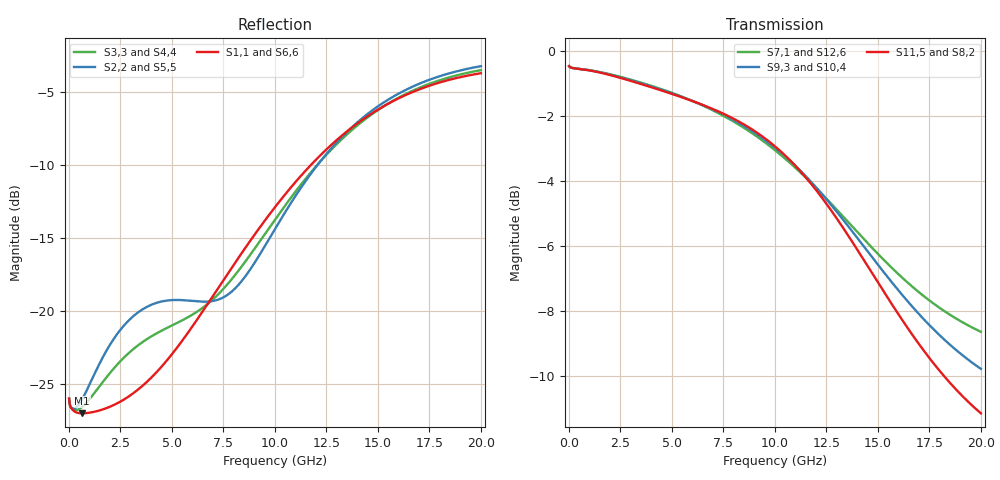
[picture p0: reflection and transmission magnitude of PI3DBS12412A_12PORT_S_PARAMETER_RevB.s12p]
! NPort=12 DATA=2000 NOISE=0 GROUPDELAY=0 COMPLEX_DATAFORMAT=POLAR
! NumOfBlock=1 NumOfParam=0
! .MODEL Smodel S TSTONEFILE=PI3DBS12412A_12PORT_S_PARAMETER_RevB.s12p TYPE=S
!  -- The above .MODEL line can be used for the S element in the netlist.
!  Port definition:
!  Port1 = INPUT1+
!  Port2 = INPUT1-
!  Port3 = INPUT2+
!  Port4 = INPUT2-
!  Port5 = INPUT3+
!  Port6 = INPUT3-
!  Port7 = OUTPUT1+
!  Port8 = OUTPUT1-
!  Port9 = OUTPUT2+
!  Port10 = OUTPUT2-
!  Port11 = OUTPUT3+
!  Port12 = OUTPUT3-
# Hz S MA R  50
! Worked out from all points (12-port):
!   2000 points, 10 MHz to 20 GHz, reference 50 ohm
!   strongest paths, dB at 10 MHz, 5.01 GHz, 10.01 GHz, 15.01 GHz, 20 GHz:
!     S11,5: -0.5, -1.3, -2.9, -7.1, -11.2
!     S8,2: -0.5, -1.3, -2.9, -7.1, -11.2
!     S9,3: -0.5, -1.3, -3.0, -6.6, -9.8
!     S10,4: -0.5, -1.3, -3.0, -6.6, -9.8
!     S7,1: -0.5, -1.3, -3.1, -6.3, -8.6
!     S12,6: -0.5, -1.3, -3.1, -6.3, -8.6
!   lowest |S11| = -27.0 dB at 650 MHz (marker M1), VSWR 1.09, Z = 54 - j2.3 ohm
!   |S11| at or under -10 dB: start of sweep to 11.75 GHz
